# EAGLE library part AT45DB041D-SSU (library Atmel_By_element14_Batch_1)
4-megabit DataFlash
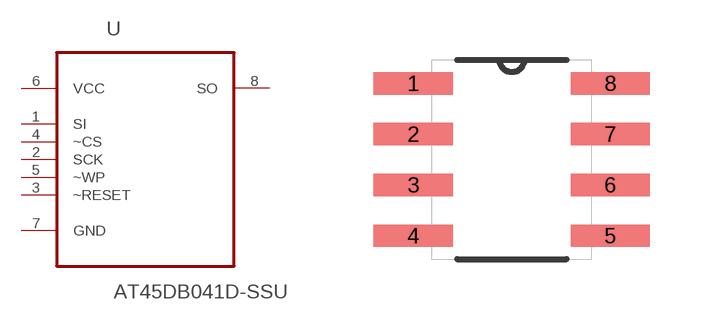
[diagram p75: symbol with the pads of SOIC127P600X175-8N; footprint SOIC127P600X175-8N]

Designator prefix U

## AT45DB041D-SSU (MPN: AT45DB041D-SSU; OC_FARNELL: 1455037; OC_NEWARK: 58M3835; PACKAGE: SOIC-8; SUPPLIER: Atmel)  [SOIC127P600X175-8N]
1  SI  in
2  SCK  in
3  ~RESET  in
4  ~CS  in
5  ~WP  in
6  VCC  pwr
7  GND  pas
8  SO  out

## Footprint SOIC127P600X175-8N (pad centres in mm)
smd 1.981 x 0.559: 1 -2.464,1.905; 2 -2.464,0.635; 3 -2.464,-0.635; 4 -2.464,-1.905; 5 2.464,-1.905; 6 2.464,-0.635; 7 2.464,0.635; 8 2.464,1.905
